(* Logix 5000 AddOnInstructionDefinition export AMCI_5034_PTO_AM_MAM; software revision 37.00 *)

TYPE AMCI_5034_PTO_AM_Input_Data :
STRUCT
   ConnectionFaulted : DINT;
   MovingCW : BOOL;
   MovingCCW : BOOL;
   InHoldState : BOOL;
   Stopped : BOOL;
   AtHome : BOOL;
   Accelerating : BOOL;
   Decelerating : BOOL;
   MoveComplete : BOOL;
   HomeInvalid : BOOL;
   InvalidProfile : BOOL;
   PositionInvalid : BOOL;
   InputError : BOOL;
   CommandError : BOOL;
   ConfigurationError : BOOL;
   ModuleOK : BOOL;
   GeneralPurposeOutputStatus : BOOL;
   Input1Active : BOOL;
   Input2Active : BOOL;
   Input3Active : BOOL;
   Input4Active : BOOL;
   bit_20_reserved : BOOL;
   bit_21_reserved : BOOL;
   bit_22_reserved : BOOL;
   EncoderFollowerMode : BOOL;
   BlendMoveRunning : BOOL;
   BlendMoveAcknowledge : BOOL;
   MinimumRegistrationProgrammed : BOOL;
   EncoderMotionDirection : BOOL;
   MultipleInputsWithSameFunction : BOOL;
   FSCExceedsNumberOfDataBits : BOOL;
   AbsoluteEncoderSetupError : BOOL;
   bit_31_reserved : BOOL;
   CurrentPosition : DINT;
   EncoderPosition : DINT;
   CapturedPosition : DINT;
END_STRUCT
END_TYPE

TYPE AMCI_5034_PTO_AM_Output_Data :
STRUCT
   Command_Word : DINT;
   TargetPosition : DINT;
   TargetVelocity : UDINT;
   Acceleration : DINT;
   Deceleration : DINT;
END_STRUCT
END_TYPE

ADD_ON_INSTRUCTION AMCI_5034_PTO_AM_MAM   (* revision 1.0, vendor AMCI, ExecuteEnableInFalse *)
// Absolute and Relative Moves
// Revision note:
// V1.0 10/01/2025 Initial release of AOI
// Help:
// MOTION AXIS MOVE: Performs Absolute or Relative Moves
// AXIS INPUT DATA:  Input data from the AMCI 5034-PTO-AM.   Uses the AMCI_5034_PTO_Input_Data User Defined Data Type.
// AXIS OUTPUT DATA; Output data from the AOI to the AMCI 5034-PTO-AM.    Uses the AMCI_5034_PTO_Output_Data User Defined Data Type.
// MOVE TYPE: 0 = Absolute Move, 1 = Relative Move
// TARGETPOSITION: Target Position of the Absolute Move or the distance to move of a Relative                                             Move.
// TARGETVELOCITY: Speed of move in units of steps / sec
// ACCELERATION: Acceleration Rate in units of steps / sec / ms
// DECELERATION:  Deceleration Rate in units of steps / sec / ms
// EN (Enable) Set when rung is true, Reset when rung is false
// DN (Done) Set when command is sent to the motion device.  Reset when the rung is false.
// ER (Error) Set when a command or input error failed to clear.  Reset when the rung is false.
// IP (In Process) Set when motion is occurring.   Reset when motion stops or the rung goes false.
// PC (Process Complete) Set when the move is complete.  Reset the next time the rung with the AOI transitions                                       from False to True.
VAR_IN_OUT
   Axis_Input_Data : AMCI_5034_PTO_AM_Input_Data; {required}
   Axis_Output_Data : AMCI_5034_PTO_AM_Output_Data; {required}
END_VAR
VAR_INPUT
   Move_type_0_Absolute_1_Relative : BOOL; {required}   // 0=absolute 1=relative
   _0_normal_1_S_Curve_Acceleration : BOOL;
   _0_Triangular_1_Trapezoidal_S_Curve : BOOL;
   TargetPosition : DINT; {required}
   TargetVelocity : DINT; {required}
   Acceleration : DINT; {required}
   Deceleration : DINT; {required}
END_VAR
VAR_OUTPUT
   EN : BOOL; {visible}   // set when rung with AOI is true
   DN : BOOL; {access Read Only, visible}   // set when move was succesfully initiated
   ER : BOOL; {visible}   // set when input error, command error, or configuration error
   IP : BOOL; {visible}   // set when motion occurring
   PC : BOOL; {visible}   // set when process complete
END_VAR
VAR
   command_data_block : DINT[5];
        [0]   // Command Word
        [1]   // Target Position
        [2]   // Programmed Speed
        [3]   // Acceleration
        [4]   // Deceleration
   motion_occurring : BOOL; {access None}
   Internal_Enable : BOOL; {access None}   // set when driver ready to receive motion command
END_VAR

ROUTINE EnableInFalse   (* ladder *)
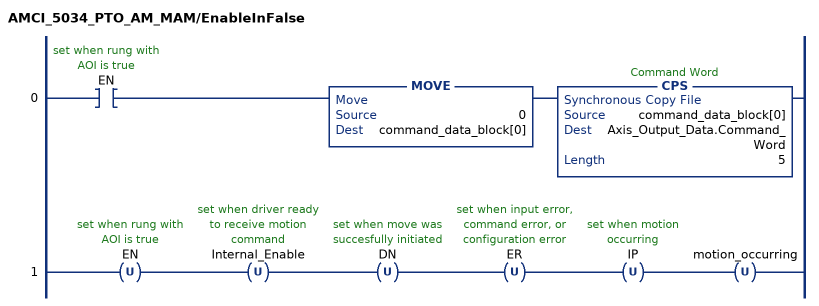
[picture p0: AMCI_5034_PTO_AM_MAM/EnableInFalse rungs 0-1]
   0: XIC(EN)MOVE(0,command_data_block[0])CPS(command_data_block[0],Axis_Output_Data.Command_Word,5);
   1: OTU(EN)OTU(Internal_Enable)OTU(DN)OTU(ER)OTU(IP)OTU(motion_occurring);
END_ROUTINE

ROUTINE Logic   (* ladder *)
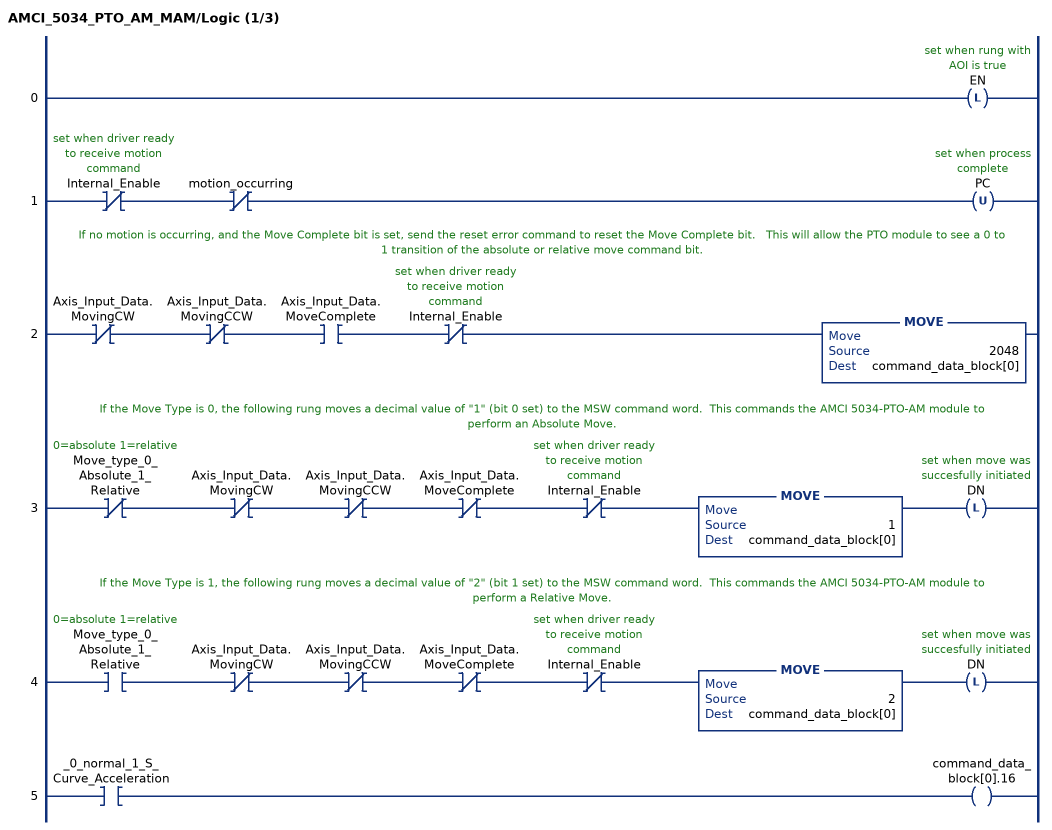
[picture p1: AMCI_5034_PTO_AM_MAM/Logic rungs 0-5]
   0: OTL(EN);
   1: XIO(Internal_Enable)XIO(motion_occurring)OTU(PC);
   // If no motion is occurring, and the Move Complete bit is set, send the reset error command to reset the Move Complete bit.   This will allow the PTO module to see a 0 to 1 transition of the absolute or relative move command bit.
   2: XIO(Axis_Input_Data.MovingCW)XIO(Axis_Input_Data.MovingCCW)XIC(Axis_Input_Data.MoveComplete)XIO(Internal_Enable)MOVE(2048,command_data_block[0]);
   // If the Move Type is 0, the following rung moves a decimal value of "1" (bit 0 set) to the MSW command word.  This commands the AMCI 5034-PTO-AM module to perform an Absolute Move.
   3: XIO(Move_type_0_Absolute_1_Relative)XIO(Axis_Input_Data.MovingCW)XIO(Axis_Input_Data.MovingCCW)XIO(Axis_Input_Data.MoveComplete)XIO(Internal_Enable)MOVE(1,command_data_block[0])OTL(DN);
   // If the Move Type is 1, the following rung moves a decimal value of "2" (bit 1 set) to the MSW command word.  This commands the AMCI 5034-PTO-AM module to perform a Relative Move.
   4: XIC(Move_type_0_Absolute_1_Relative)XIO(Axis_Input_Data.MovingCW)XIO(Axis_Input_Data.MovingCCW)XIO(Axis_Input_Data.MoveComplete)XIO(Internal_Enable)MOVE(2,command_data_block[0])OTL(DN);
   5: XIC(_0_normal_1_S_Curve_Acceleration)OTE(command_data_block[0].16);
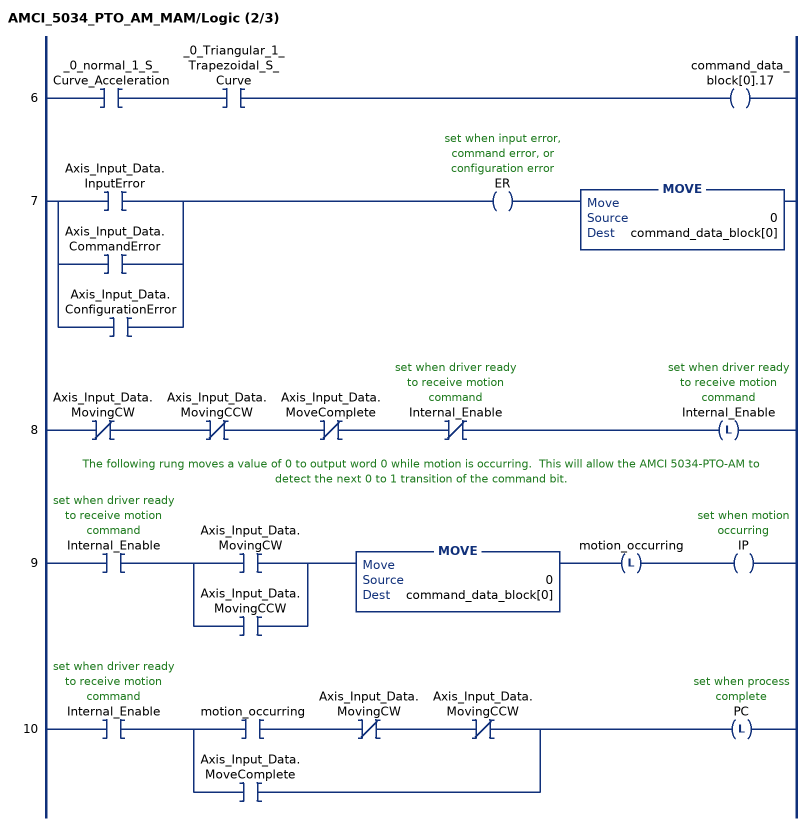
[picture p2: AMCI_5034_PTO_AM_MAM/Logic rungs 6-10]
   6: XIC(_0_normal_1_S_Curve_Acceleration)XIC(_0_Triangular_1_Trapezoidal_S_Curve)OTE(command_data_block[0].17);
   7: [XIC(Axis_Input_Data.InputError) ,XIC(Axis_Input_Data.CommandError) ,XIC(Axis_Input_Data.ConfigurationError) ]OTE(ER)MOVE(0,command_data_block[0]);
   8: XIO(Axis_Input_Data.MovingCW)XIO(Axis_Input_Data.MovingCCW)XIO(Axis_Input_Data.MoveComplete)XIO(Internal_Enable)OTL(Internal_Enable);
   // The following rung moves a value of 0 to output word 0 while motion is occurring.  This will allow the AMCI 5034-PTO-AM to detect the next 0 to 1 transition of the command bit.
   9: XIC(Internal_Enable)[XIC(Axis_Input_Data.MovingCW) ,XIC(Axis_Input_Data.MovingCCW) ]MOVE(0,command_data_block[0])OTL(motion_occurring)OTE(IP);
   10: XIC(Internal_Enable)[XIC(motion_occurring) XIO(Axis_Input_Data.MovingCW) XIO(Axis_Input_Data.MovingCCW) ,XIC(Axis_Input_Data.MoveComplete) ]OTL(PC);
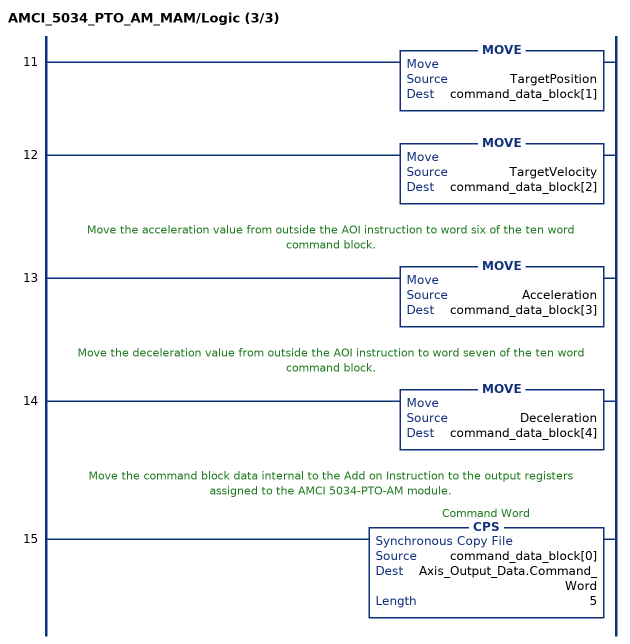
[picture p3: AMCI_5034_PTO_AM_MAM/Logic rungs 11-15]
   11: MOVE(TargetPosition,command_data_block[1]);
   12: MOVE(TargetVelocity,command_data_block[2]);
   // Move the acceleration value from outside the AOI instruction to word six of the ten word command block.
   13: MOVE(Acceleration,command_data_block[3]);
   // Move the deceleration value from outside the AOI instruction to word seven of the ten word command block.
   14: MOVE(Deceleration,command_data_block[4]);
   // Move the command block data internal to the Add on Instruction to the output registers assigned to the AMCI 5034-PTO-AM module.
   15: CPS(command_data_block[0],Axis_Output_Data.Command_Word,5);
END_ROUTINE
END_ADD_ON_INSTRUCTION
